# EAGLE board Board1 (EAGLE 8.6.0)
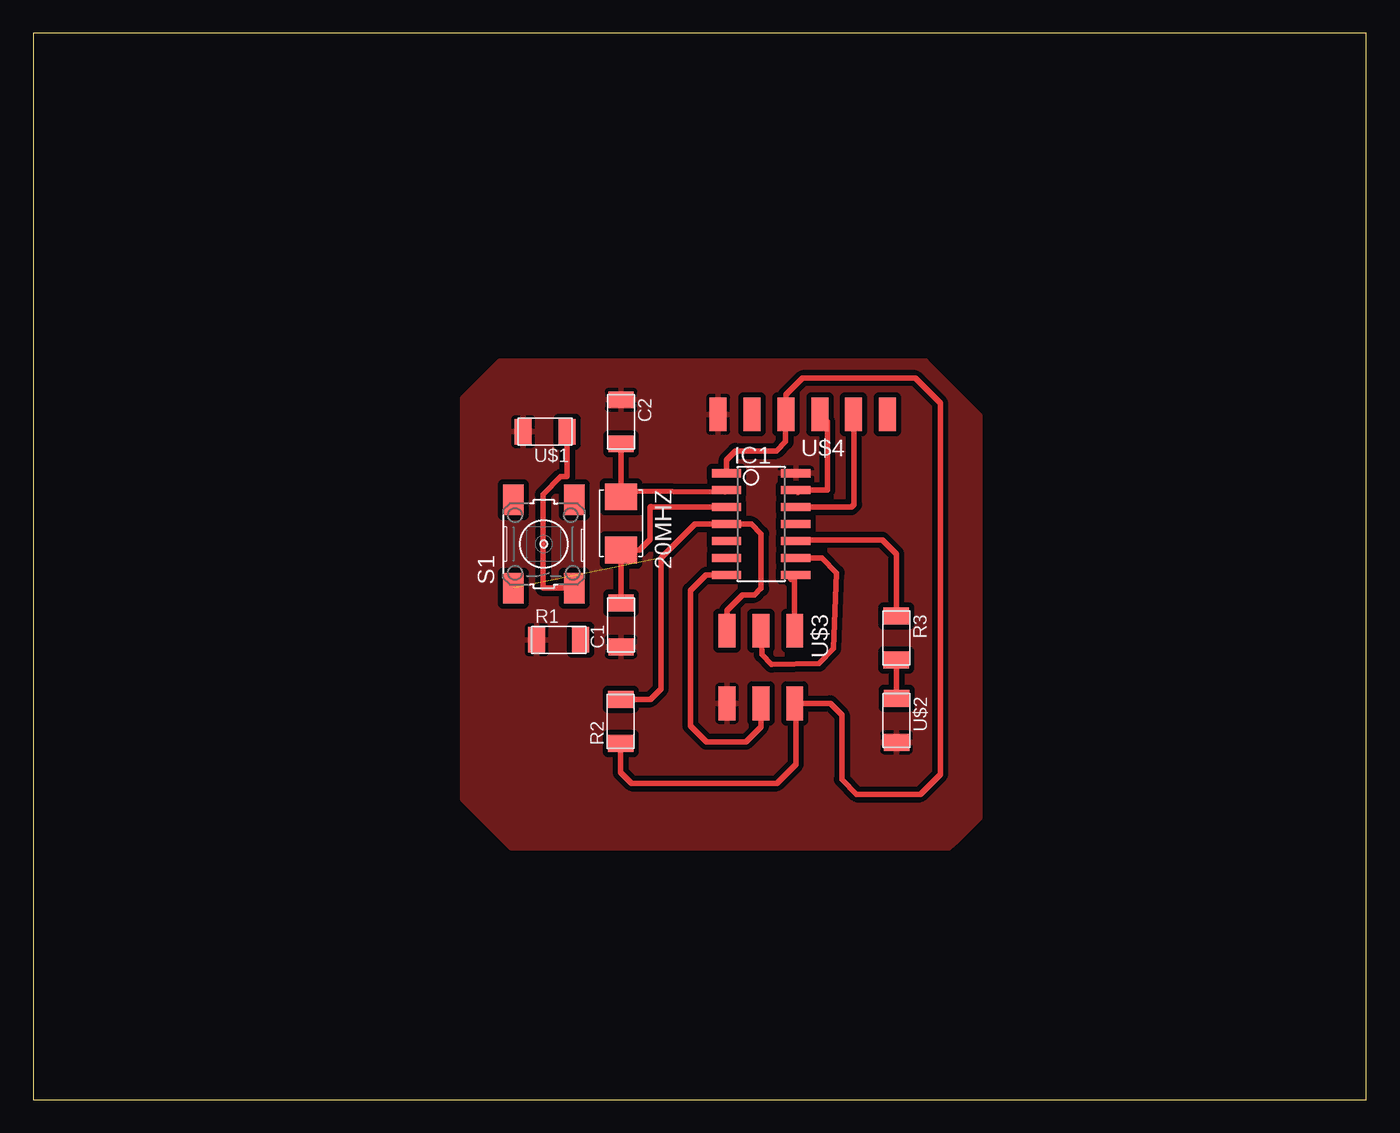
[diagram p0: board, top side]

Size 100 x 80 mm. Coordinates in mm from the lower left corner, seen from the top.
Outline: 0,0 100,0 100,80 0,80 0,0
Copper layers (1*16): Top 0.035mm / dielectric 1.5mm / Bottom 0.035mm
Design rules "aa *": minimum track width 10mil, minimum drill 0.4mm, track to track 0.4mm, track to pad 0.4mm, pad to pad 0.42mm, via to via 0.42mm, smd to smd 0.42mm, copper to edge 40mil, drill to drill 0.8mm, minimum pad ring 10mil, minimum via ring 8mil, stop-mask expansion 4mil, vias tented up to drill 0mil, thermal gap 10mil

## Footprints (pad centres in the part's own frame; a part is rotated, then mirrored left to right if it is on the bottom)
2-SMD-5X3MM = smd 2 x 2.4: P$1 -2,0; P$2 2,0
C1206FAB = smd 1.27 x 1.905: 1 -1.651,0; 2 1.651,0
SOIC14 = smd 0.61 x 2.21: 1 -3.81,-2.603; 2 -2.54,-2.603; 3 -1.27,-2.603; 4 0,-2.603; 5 1.27,-2.603; 6 2.54,-2.603; 7 3.81,-2.603; 8 3.81,2.603; 9 2.54,2.603; 10 1.27,2.603; 11 0,2.603; 12 -1.27,2.603; 13 -2.54,2.603; 14 -3.81,2.603
R1206FAB = smd 1.27 x 1.905: 1 -1.651,0; 2 1.651,0
6MM_SWITCH = smd 2.286 x 1.524: 1 -3.302,2.286; 2 3.302,2.286; 3 -3.302,-2.286; 4 3.302,-2.286
LED1206FAB = smd 1.27 x 1.905: 1 -1.651,0; 2 1.651,0
2X03SMD = smd 2.54 x 1.27: 1 -2.54,2.54; 2 2.92,2.54; 3 -2.54,0; 4 2.92,0; 5 -2.54,-2.54; 6 2.92,-2.54
1X06SMD = smd 2.54 x 1.27: 1 0,6.35; 2 0,3.81; 3 0,1.27; 4 0,-1.27; 5 0,-3.81; 6 0,-6.35

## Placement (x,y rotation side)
20MHZ  CRYSTAL  [2-SMD-5X3MM]  44.09,43.23 270 top
C1  10 pF  [C1206FAB]  44.09,35.61 90 top
C2  10 pF  [C1206FAB]  44.09,50.85 270 top
IC1  ATTINY44-SSU  [SOIC14]  54.61,43.18 270 top
R1  499  [R1206FAB]  39.42,34.49 0 top
R2  10 k  [R1206FAB]  44.07,28.37 90 top
R3  499  [R1206FAB]  64.74,34.62 270 top
S1  [6MM_SWITCH]  38.3,41.68 90 top
U$1  LEDFAB1206  [LED1206FAB]  38.4,50.11 180 top
U$2  LEDFAB1206  [LED1206FAB]  64.77,28.45 270 top
U$3  AVRISPSMD  [2X03SMD]  54.58,32.64 270 top
U$4  FTDI-SMD-HEADER  [1X06SMD]  57.73,51.41 90 top

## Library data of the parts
20MHZ C1 C2 IC1 R1-R3 S1 U$1-U$4 = fab (1)

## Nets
CTS: U$4.2
GND: C1.1 C2.1 IC1.14 R1.1 U$1.2 U$2.2 U$3.6 U$4.1
LED: IC1.10 R3.1
MISO: IC1.8 U$3.1
MOSI: IC1.7 U$3.4
N$1: R3.2 U$2.1
N$2: S1.3 U$1.1
N$3: R1.2
RST: IC1.4 R2.2 S1.1 U$3.5
RTS: U$4.6
RXD: IC1.12 U$4.5
SCK: IC1.9 U$3.3
TXD: IC1.13 U$4.4
VCC: IC1.1 R2.1 U$3.2 U$4.3
XTA1: 20MHZ.P$1 C2.2 IC1.2
XTA2: 20MHZ.P$2 C1.2 IC1.3

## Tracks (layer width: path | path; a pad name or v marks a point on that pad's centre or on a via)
GND
  pour Top: 66.98,55.4 35.03,55.4 32.21,52.58 32.21,22.56 35.89,18.87 68.71,18.87 69.14,19.3 71.02,21.18 71.02,23.24 71.02,51.28 66.98,55.32
LED
  Top 0.406: R3.1 64.75,40.95 63.7,41.99 57.29,41.99 IC1.10
MISO
  Top 0.406: 56.84,39 IC1.8 57.12,39.28 U$3.1
MOSI
  Top 0.406: U$3.4 54.59,27.96 53.47,26.85 50.49,26.85 49.3,28.04 49.3,38.2 50.47,39.37 IC1.7
N$1
  Top 0.406: R3.2 U$2.1
N$2
  Top 0.406: U$1.1 40.06,46.78 40.01,46.73 39.57,46.73 38.23,45.39 38.23,38.43 38.28,38.38 S1.3
RST  (1 unrouted)
  Top 0.406: 44.07,30.33 R2.2 | 44.12,29.97 R2.2 | R2.2 46.3,30.02 47.09,30.81 47.09,40.62 49.66,43.18 IC1.4 53.87,43.18 54.61,42.44 54.61,38.33 54.56,38.33 54.1,37.87 53.21,37.87 52.05,36.7 U$3.5
RXD
  Top 0.406: 57.31,44.35 IC1.12 61.37,44.45 61.57,44.65 61.57,51.38 U$4.5
SCK
  Top 0.406: U$3.3 54.66,33.38 55.4,32.64 58.95,32.72 60.02,33.83 60.27,39.52 59.16,40.64 IC1.9
TXD
  Top 0.406: 57.38,45.56 IC1.13 59.56,45.72 59.56,50.85 U$4.4
VCC
  Top 0.406: 51.93,47.07 IC1.1 52.01,47.99 52.68,48.67 55.75,48.67 56.44,49.35 56.44,51.84 56.46,51.87 | 56.46,51.87 56.46,52.88 57.71,54.13 66.17,54.13 68.05,52.25 68.05,24.41 66.55,22.91 61.77,22.91 60.66,24.03 60.66,28.85 59.79,29.72 U$3.2 57.2,29.64 57.2,25.15 55.78,23.72 44.88,23.72 44.07,24.54 R2.1 | 56.46,51.87 U$4.3
XTA1
  Top 0.406: 20MHZ.P$1 44.09,45.64 | 44.09,45.64 C2.2 | IC1.2 51.88,45.59 44.09,45.64
XTA2
  Top 0.406: C1.2 20MHZ.P$2 45.47,41.23 46.28,42.04 46.28,44.42 46.35,44.5 46.41,44.45 IC1.3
